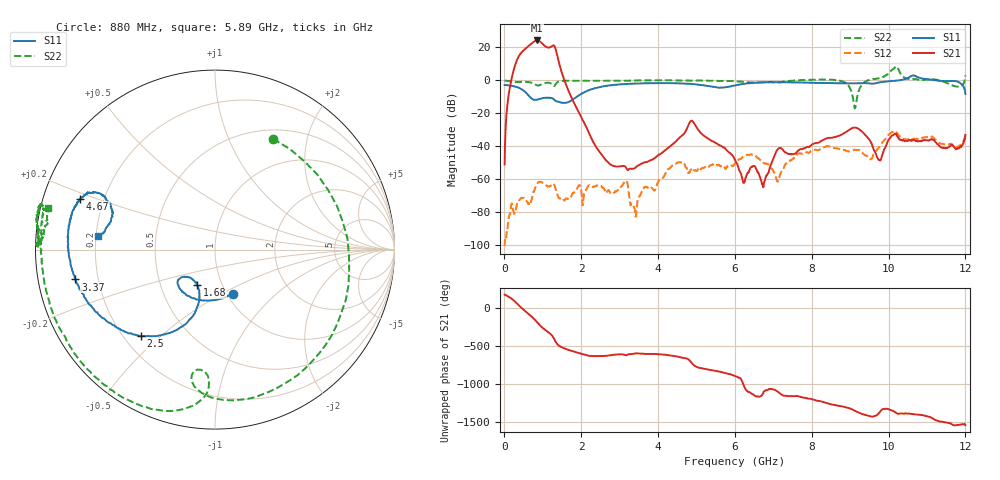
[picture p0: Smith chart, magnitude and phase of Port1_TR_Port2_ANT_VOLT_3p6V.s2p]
! Created Mon Aug 25 11:00:22 2025
# hz S ma R 50
! 2 Port Network Data from SP1.SP block
! freq  magS11  angS11  magS21  angS21  magS12  angS12  magS22  angS22
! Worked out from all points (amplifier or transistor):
!   1200 points, 10 MHz to 12 GHz, reference 50 ohm
!   highest |S21| = 24.2 dB at 860 MHz (marker M1)
!   |S21| within 3 dB of that: 650.8 MHz to 1.038 GHz (387.7 MHz wide, 45.9 % of centre)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
!   unconditionally stable (mu >= 1): start of sweep to 3.537 GHz; 4.513 GHz to 7.63 GHz; 8.676 GHz to 9.465 GHz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
!   at 2.01 GHz: K = 855.86, MAG = -9.7 dB, |S12| = -67.9 dB
!   at 6.01 GHz: K = 2582.46, MAG = -36.3 dB, |S12| = -50.1 dB
!   at 12 GHz: K = -802.18, MSG = -0.3 dB, |S12| = -32.4 dB
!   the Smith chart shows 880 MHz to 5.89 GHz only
!   S11 on the Smith chart (normalised r, x): 880 MHz: 1.07, -0.56; 1.68 GHz: 0.76, -0.32; 2.5 GHz: 0.27, -0.43; 3.37 GHz: 0.12, -0.10; 4.67 GHz: 0.11, +0.18; 5.89 GHz: 0.21, +0.06
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1e7  0.7209 178.6  0.002846 172.2  9.531e-06 -172.4  0.9837 176.3
3.5e8  0.6164 126.3  4.605 45.8  0.0001938 127.0  0.8935 2.3
5.2e8  0.4714 85.1  8.446 -34.1  0.0002621 82.7  0.9061 -99.2
7.1e8  0.2849 9.0  13.07 -114.7  0.0002402 117.4  0.8456 -178.7
8e8  0.2557 -34.9  15.48 -158.8  0.0005322 107.3  0.7556 128.4
8.6e8  0.2608 -61.1  16.16 168.1  0.0007513 86.6  0.7014 79.9
8.8e8  0.2655 -68.0  16.02 156.9  0.0008114 77.5  0.6966 62.3
1e9  0.2887 -100.6  12.55 95.9  0.0007862 31.7  0.7859 -25.9
1.22e9  0.2925 -132.2  10.4 9.3  0.0006591 -26.5  0.8013 -95.4
1.33e9  0.2432 -140.3  9.426 -78.5  0.0005657 -111.8  0.7354 -92.5
1.41e9  0.226 -137.6  4.015 -129.4  0.0002901 -157.8  0.9148 -102.5
1.68e9  0.2232 -116.7  0.4598 167.4  0.000255 140.1  0.9746 -130.7
2.01e9  0.3924 -108.5  0.0735 118.1  0.0004039 61.3  0.9695 -151.7
2.5e9  0.6351 -130.7  0.00635 87.9  0.0006524 55.3  0.9677 -175.5
3.37e9  0.7954 -167.9  0.002127 118.2  0.0001517 4.9  0.9898 165.9
4.01e9  0.8237 172.9  0.005458 112.3  0.0008682 75.2  1.01 167.4
4.67e9  0.8016 159.3  0.02363 62.7  0.003127 -24.9  0.9923 174.4
5.89e9  0.6558 173.3  0.006058 -151.0  0.00256 -16.0  0.9606 166.1
6.01e9  0.7046 175.8  0.00381 -174.7  0.003118 -5.7  0.9371 159.4
8.01e9  0.8431 159.4  0.01141 -114.7  0.007712 -92.8  1.042 56.3
1.001e10  0.9382 127.8  0.01638 110.9  0.0229 132.9  1.667 137.2
1.2e10  0.3887 75.3  0.02233 -96.1  0.02408 -85.1  1.42 64.6
